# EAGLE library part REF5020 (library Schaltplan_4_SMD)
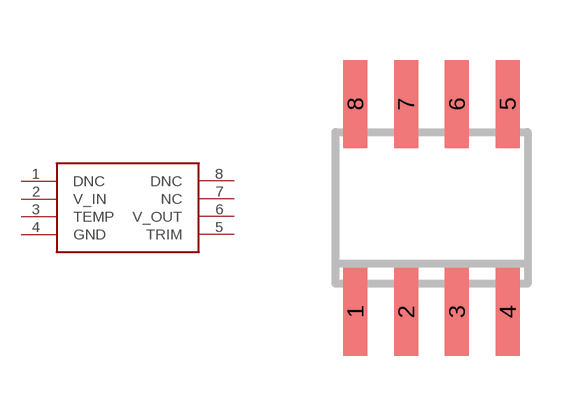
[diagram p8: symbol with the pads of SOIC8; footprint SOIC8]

Designator prefix -

## REF5020  [SOIC8]
1  DNC
2  V_IN
3  TEMP
4  GND
5  TRIM
6  V_OUT
7  NC
8  DNC

## Footprint SOIC8 (pad centres in mm)
Small Outline IC
smd 0.6 x 2.2: 1 -1.905,-2.6; 2 -0.635,-2.6; 3 0.635,-2.6; 4 1.905,-2.6; 5 1.905,2.6; 6 0.635,2.6; 7 -0.635,2.6; 8 -1.905,2.6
